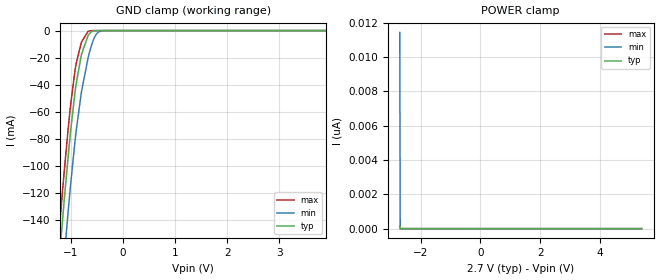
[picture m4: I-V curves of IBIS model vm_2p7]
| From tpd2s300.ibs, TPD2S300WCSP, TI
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|   VM_2p7 Model
[Model]   vm_2p7
Model_type   Input
Vinl = 0.81
Vinh = 1.89
|   typ   min   max
C_comp   15.3335pF   10.9389pF   19.9888pF
[Model spec]
|subparameter
Vinl   0.81   0.8097   0.8103
Vinh   1.89   1.8893   1.8907
| Where nom  PVT is Nominal Process, 2.7V, 27C
|   Fast PVT is Strong Process,  2.701V, -40C
|   Slow PVT is Weak Process,   2.699V, 125C
[Voltage Range]   2.7   2.699   2.701
[Temperature Range]   27   125   -40
[Power Clamp Reference]   2.7   2.699   2.701
[GND Clamp Reference]   0   0   0
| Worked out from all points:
|   GND clamp passes 1 mA (typ) near -0.60 V on its own axis
[GND Clamp]
|   Voltage   I(typ)   I(min)   I(max)
-2.7V     -930.6mA   -1.012A    -893.5mA
-1.331V   -223.8mA   -269.8mA   -201.1mA
-1.21V    -165.5mA   -209.2mA   -143.6mA
-1.193V   -157.9mA   -201.4mA   -136.1mA
-1.112V   -121.1mA   -163.1mA   -99.91mA
-1.048V   -93.33mA   -134.1mA   -72.98mA
-918mV    -46.38mA   -82.64mA   -30.15mA
-796.5mV  -18.57mA   -46.47mA   -9.071mA
-658.8mV  -3.407mA   -19.25mA   -568.9uA
-529.2mV  -101.5uA   -4.076mA   -7.996uA
-375.3mV  -345.2nA   -122.5uA   0A
5.4V      0A         0A         0A
[POWER Clamp]
|   Voltage   I(typ)   I(min)   I(max)
-2.7V     152.2pA    11.43nA    123.2pA
-2.684V   0A         0A         0A
-2.676V   0A         0A         0A
5.4V      0A         0A         0A
